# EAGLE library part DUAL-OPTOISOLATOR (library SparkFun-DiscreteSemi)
Optocoupler, Phototransistor Output, Dual Channel Optically coupled pairs with a gallium arsenide infrared LED and a silicon NPN phototransistor. Signal information, including a DC level, can be transmitted by the device while maintaining a high degree of electrical isolation between input and output. Datasheet SparkFun Products: SparkFun Opto-isolator Breakout
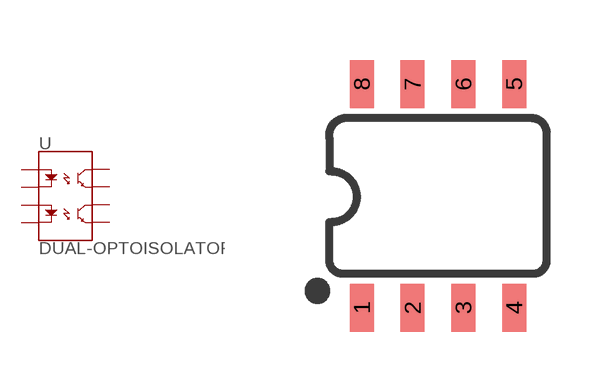
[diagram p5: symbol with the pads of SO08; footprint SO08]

Designator prefix U

## DUAL-OPTOISOLATOR_SOIC8 (PROD_ID: IC-09076)  [SO08]
1  A1
2  C1
3  A2
4  C2
5  EM2
6  CL2
7  EM1
8  CL1

## Footprint SO08 (pad centres in mm)
SOIC, 0.15 inch width
smd 0.6 x 1.2: 1 -1.905,-2.8; 2 -0.635,-2.8; 3 0.635,-2.8; 4 1.905,-2.8; 5 1.905,2.8; 6 0.635,2.8; 7 -0.635,2.8; 8 -1.905,2.8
